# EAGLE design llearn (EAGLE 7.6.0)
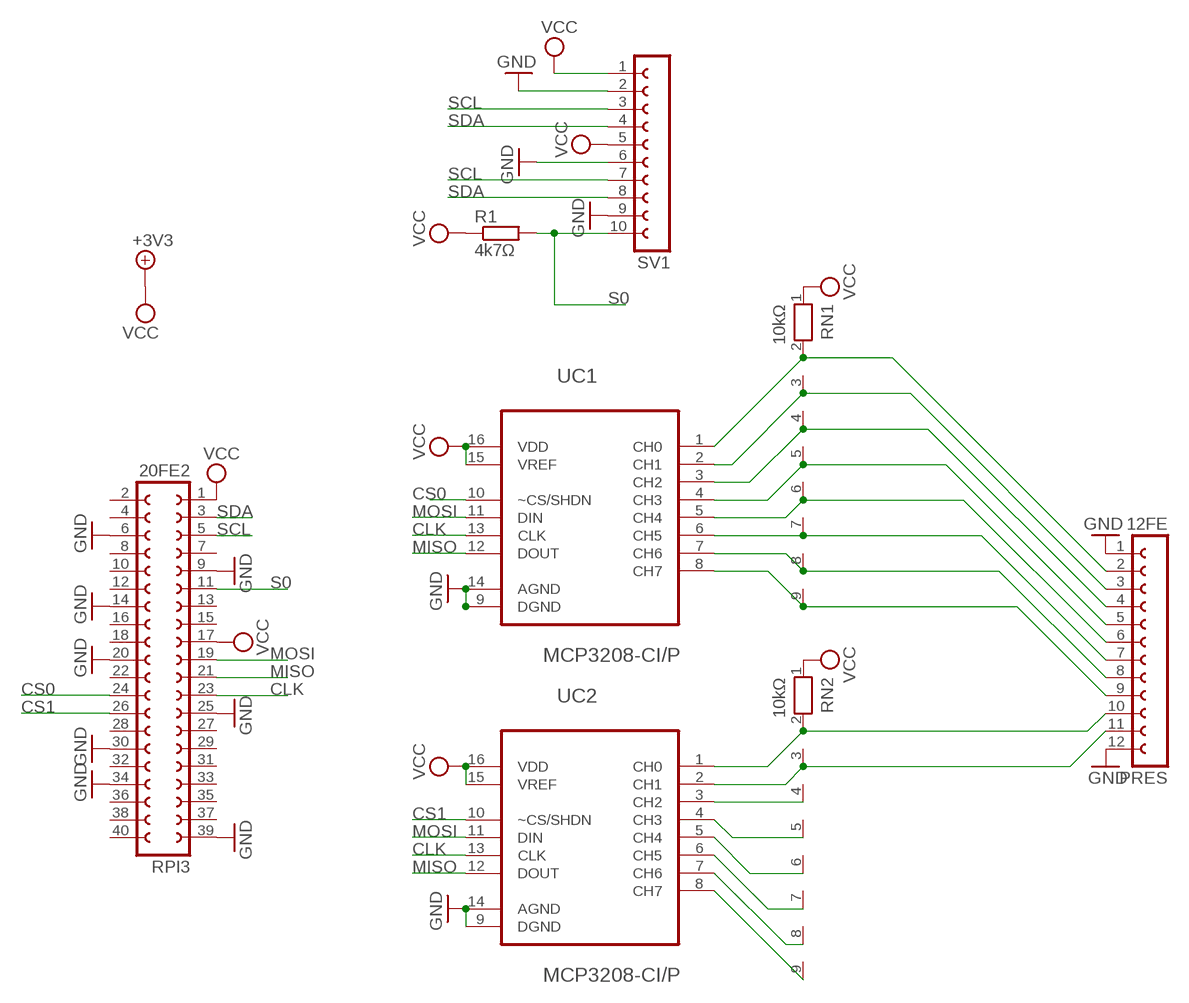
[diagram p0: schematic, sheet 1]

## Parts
PRES  12FE  FE12-1  [FE12]
R1  4k7Ω  R-EU_0207/10  [0207/10]
RN1  10kΩ  RN08  [RN-9]
RN2  10kΩ  RN08  [RN-9]
RPI3  20FE2  FE20-2  [FE20-2]
SV1  FE10-1  [FE10]
UC1  MCP3208-CI/P  [DIP254P762X432-16]
UC2  MCP3208-CI/P  [DIP254P762X432-16]

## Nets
CLK: RPI3.23 UC1.13(CLK) UC2.13(CLK)
CS0: RPI3.24 UC1.10(~CS/SHDN)
CS1: RPI3.26 UC2.10(~CS/SHDN)
GND: PRES.1 PRES.12 RPI3.6 RPI3.9 RPI3.14 RPI3.20 RPI3.25 RPI3.30 RPI3.34 RPI3.39 SV1.2 SV1.6 SV1.9 UC1.9(DGND) UC1.14(AGND) UC2.9(DGND) UC2.14(AGND)
MISO: RPI3.21 UC1.12(DOUT) UC2.12(DOUT)
MOSI: RPI3.19 UC1.11(DIN) UC2.11(DIN)
N$1: PRES.2 RN1.2 UC1.1(CH0)
N$2: PRES.3 RN1.3 UC1.2(CH1)
N$3: PRES.4 RN1.4 UC1.3(CH2)
N$4: PRES.5 RN1.5 UC1.4(CH3)
N$5: PRES.6 RN1.6 UC1.5(CH4)
N$6: PRES.7 RN1.7 UC1.6(CH5)
N$7: PRES.8 RN1.8 UC1.7(CH6)
N$8: PRES.9 RN1.9 UC1.8(CH7)
N$9: PRES.10 RN2.2 UC2.1(CH0)
N$10: PRES.11 RN2.3 UC2.2(CH1)
N$11: RN2.4 UC2.3(CH2)
N$12: RN2.5 UC2.4(CH3)
N$13: RN2.6 UC2.5(CH4)
N$14: RN2.7 UC2.6(CH5)
N$15: RN2.8 UC2.7(CH6)
N$16: RN2.9 UC2.8(CH7)
S0: R1.2 RPI3.11 SV1.10
SCL: RPI3.5 SV1.3 SV1.7
SDA: RPI3.3 SV1.4 SV1.8
VCC: R1.1 RN1.1 RN2.1 RPI3.1 RPI3.17 SV1.1 SV1.5 UC1.15(VREF) UC1.16(VDD) UC2.15(VREF) UC2.16(VDD) ; supply symbol labelled +3V3
Unconnected: RPI3.2 RPI3.4 RPI3.7 RPI3.8 RPI3.10 RPI3.12 RPI3.13 RPI3.15 RPI3.16 RPI3.18 RPI3.22 RPI3.27 RPI3.28 RPI3.29 RPI3.31 RPI3.32 RPI3.33 RPI3.35 RPI3.36 RPI3.37 RPI3.38 RPI3.40

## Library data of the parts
PRES = con-lsta:FE12-1: FEMALE HEADER; OC_FARNELL: unknown; OC_NEWARK: unknown
R1 = rcl:R-EU_: RESISTOR, European symbol
RN1 RN2 = resistor-net:RN08: RESISTOR NETWORK; OC_FARNELL: unknown; OC_NEWARK: unknown
RPI3 = con-lsta:FE20-2: FEMALE HEADER; OC_FARNELL: unknown; OC_NEWARK: unknown
SV1 = con-lsta:FE10-1: FEMALE HEADER; OC_FARNELL: unknown; OC_NEWARK: unknown
UC1 UC2 = Microchip_By_element14_Batch_1:MCP3208-CI/P: A/D Converters; MPN: MCP3208-CI/P; OC_FARNELL: 1084269; OC_NEWARK: 58K1815; PACKAGE: DIP-16; SUPPLIER: Microchip

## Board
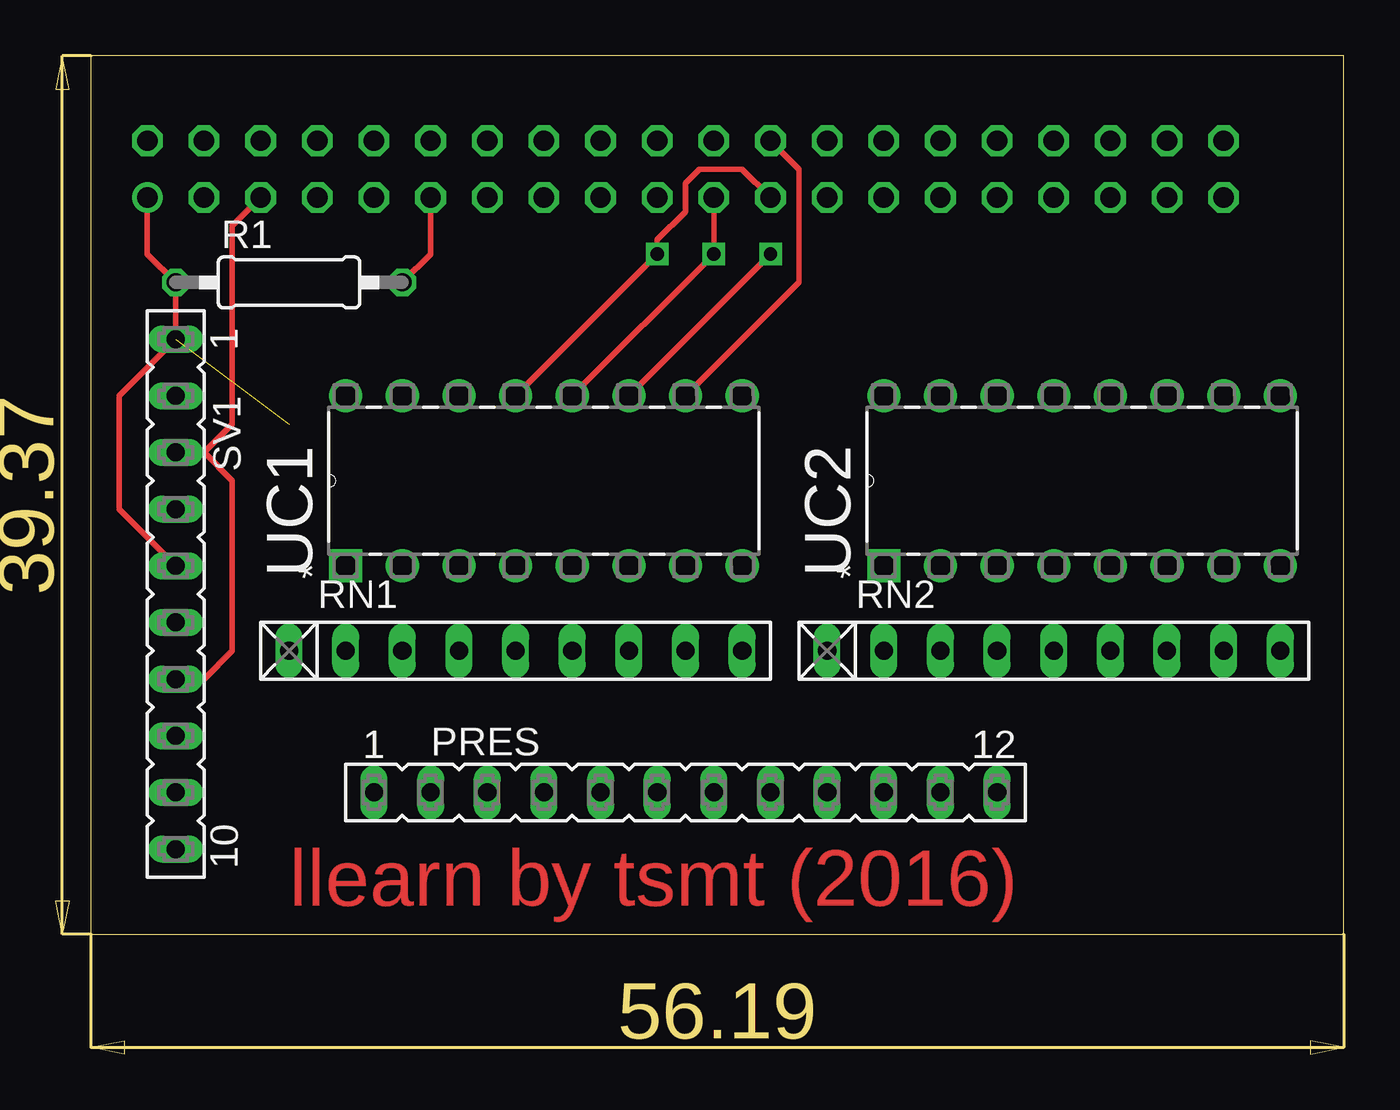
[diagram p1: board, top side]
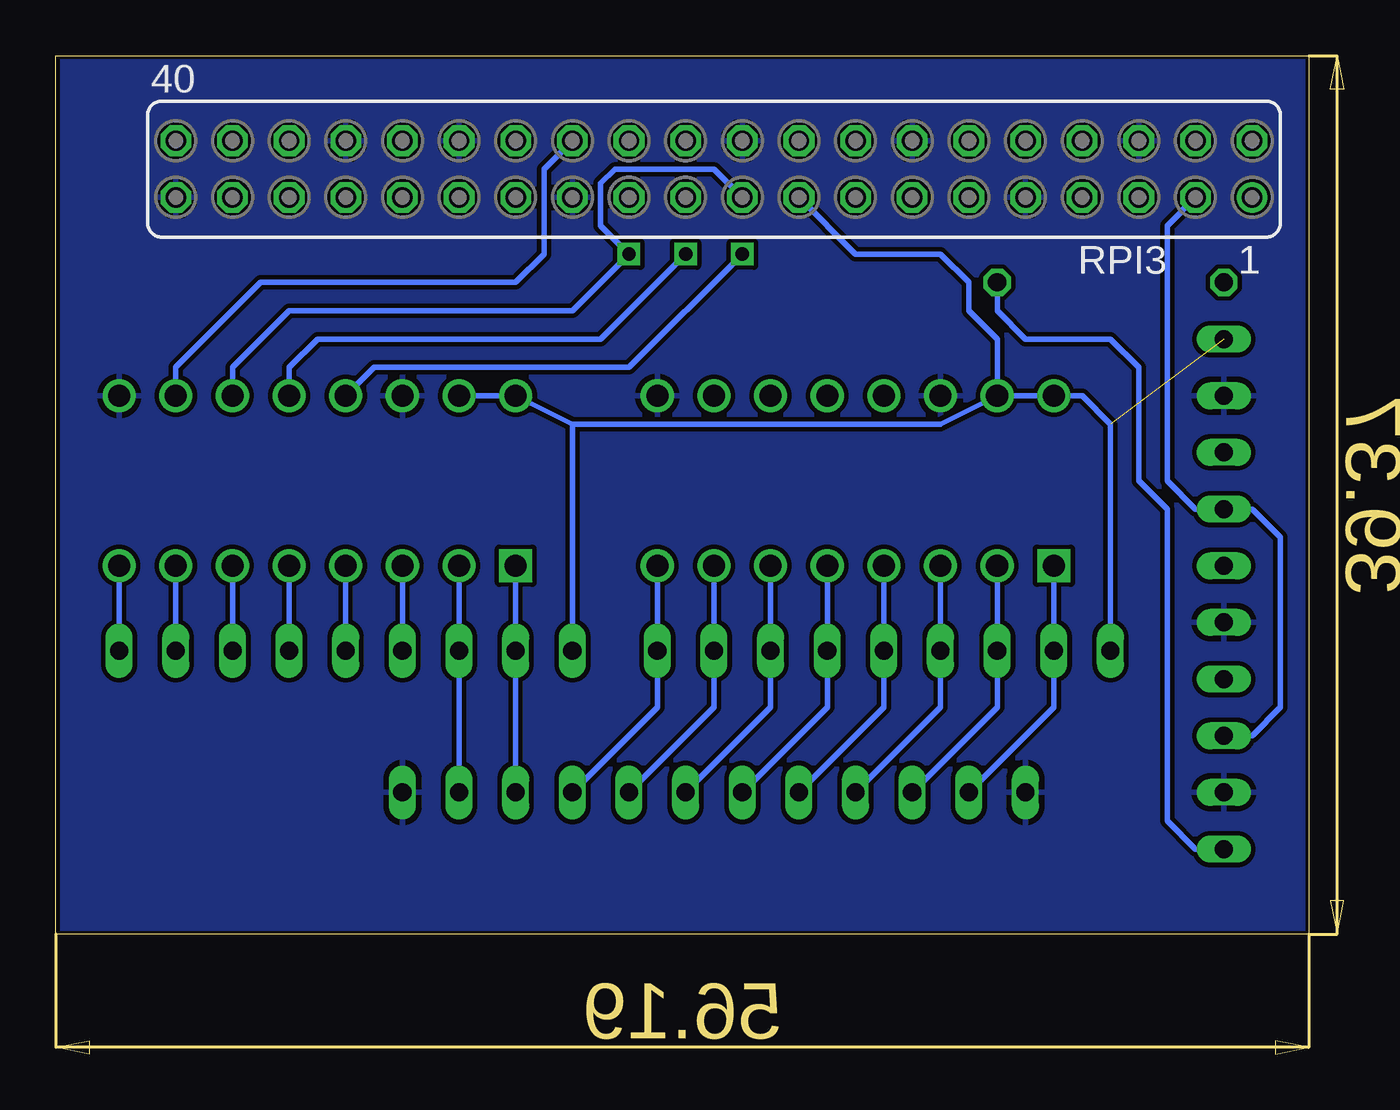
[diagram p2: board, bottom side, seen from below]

Size 57.76 x 44.75 mm. Coordinates in mm from the lower left corner, seen from the top.
Outline: 1.57,5.38 57.76,5.38 57.76,44.74 1.57,44.74 1.57,5.38
Copper layers (1*16): Top 0.035mm / dielectric 1.5mm / Bottom 0.035mm
Design rules "default *": minimum track width 0.2mm, minimum drill 0.3mm, track to track 8mil, track to pad 8mil, pad to pad 8mil, via to via 8mil, smd to smd 8mil, copper to edge 0.15mm, drill to drill 0.5mm, minimum pad ring 0.15mm, minimum via ring 8mil, stop-mask expansion 4mil, vias tented up to drill 0mil, thermal gap 10mil

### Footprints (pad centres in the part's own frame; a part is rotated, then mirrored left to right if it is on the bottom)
FE12 = drill 0.813 long: 1 -13.97,0; 2 -11.43,0; 3 -8.89,0; 4 -6.35,0; 5 -3.81,0; 6 -1.27,0; 7 1.27,0; 8 3.81,0; 9 6.35,0; 10 8.89,0; 11 11.43,0; 12 13.97,0
0207/10 = drill 0.813 octagon: 1 -5.08,0; 2 5.08,0
RN-9 = drill 0.813 long: 1 -10.16,0; 2 -7.62,0; 3 -5.08,0; 4 -2.54,0; 5 0,0; 6 2.54,0; 7 5.08,0; 8 7.62,0; 9 10.16,0
FE20-2 = drill 0.914: 1 -24.13,1.27 | drill 0.914 octagon: 2 -24.13,-1.27; 3 -21.59,1.27; 4 -21.59,-1.27; 5 -19.05,1.27; 6 -19.05,-1.27; 7 -16.51,1.27; 8 -16.51,-1.27; 9 -13.97,1.27; 10 -13.97,-1.27; 11 -11.43,1.27; 12 -11.43,-1.27; 13 -8.89,1.27; 14 -8.89,-1.27; 15 -6.35,1.27; 16 -6.35,-1.27; 17 -3.81,1.27; 18 -3.81,-1.27; 19 -1.27,1.27; 20 -1.27,-1.27; 21 1.27,1.27; 22 1.27,-1.27; 23 3.81,1.27; 24 3.81,-1.27; 25 6.35,1.27; 26 6.35,-1.27; 27 8.89,1.27; 28 8.89,-1.27; 29 11.43,1.27; 30 11.43,-1.27; 31 13.97,1.27; 32 13.97,-1.27; 33 16.51,1.27; 34 16.51,-1.27; 35 19.05,1.27; 36 19.05,-1.27; 37 21.59,1.27; 38 21.59,-1.27; 39 24.13,1.27; 40 24.13,-1.27
FE10 = drill 0.813 long: 1 -11.43,0; 2 -8.89,0; 3 -6.35,0; 4 -3.81,0; 5 -1.27,0; 6 1.27,0; 7 3.81,0; 8 6.35,0; 9 8.89,0; 10 11.43,0
DIP254P762X432-16 = drill 0.991 square: 1 -7.62,17.78 | drill 0.991: 2 -7.62,15.24; 3 -7.62,12.7; 4 -7.62,10.16; 5 -7.62,7.62; 6 -7.62,5.08; 7 -7.62,2.54; 8 -7.62,0; 9 0,0; 10 0,2.54; 11 0,5.08; 12 0,7.62; 13 0,10.16; 14 0,12.7; 15 0,15.24; 16 0,17.78

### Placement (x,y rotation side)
PRES  28.24,11.73 0 top
R1  10.46,34.59 0 top
RN1  20.62,18.08 0 top
RN2  44.75,18.08 0 top
RPI3  28.24,39.67 180 bottom
SV1  5.38,20.62 270 top
UC1  30.78,29.51 90 top
UC2  54.91,29.51 90 top

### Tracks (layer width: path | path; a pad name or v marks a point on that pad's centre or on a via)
CLK  (via drill 0.6)
  Top 0.254: RPI3.23 30.78,39.67 28.88,39.67 28.24,39.04 28.24,37.77 26.97,36.49 v26.97,35.86 UC1.13
  Bottom 0.254: v26.97,35.86 32.05,30.78 43.48,30.78 UC2.13
CS0
  Top 0.254: RPI3.24 33.32,39.67 33.32,34.59 UC1.10
CS1
  Bottom 0.254: RPI3.26 35.86,39.67 35.86,35.86 37.13,34.59 48.56,34.59 52.37,30.78 UC2.10
GND
  pour Bottom: 1.57,44.75 1.57,5.38 57.45,5.38 57.45,44.75
MISO  (via drill 0.6)
  Top 0.254: RPI3.21 v29.51,35.86 UC1.12
  Bottom 0.254: v29.51,35.86 33.32,32.05 46.02,32.05 47.29,30.78 UC2.12
MOSI  (via drill 0.6)
  Top 0.254: UC1.11 v32.05,35.86
  Bottom 0.254: RPI3.19 28.24,39.67 32.68,39.67 33.32,39.04 33.32,37.13 v32.05,35.86 34.59,33.32 47.29,33.32 49.83,30.78 UC2.11
N$1
  Bottom 0.254: UC1.1 RN1.2 13,15.54 PRES.2
N$2
  Bottom 0.254: UC1.2 RN1.3 15.54,15.54 PRES.3
N$3
  Bottom 0.254: UC1.3 RN1.4 18.08,15.54 PRES.4
N$4
  Bottom 0.254: UC1.4 RN1.5 20.62,15.54 PRES.5
N$5
  Bottom 0.254: UC1.5 RN1.6 23.16,15.54 PRES.6
N$6
  Bottom 0.254: UC1.6 RN1.7 25.7,15.54 PRES.7
N$7
  Bottom 0.254: UC1.7 RN1.8 28.24,15.54 PRES.8
N$8
  Bottom 0.254: UC1.8 RN1.9 30.78,15.54 PRES.9
N$9
  Bottom 0.254: UC2.1 RN2.2 PRES.10
N$10
  Bottom 0.254: UC2.2 RN2.3 PRES.11
N$11
  Bottom 0.254: UC2.3 RN2.4
N$12
  Bottom 0.254: UC2.4 RN2.5
N$13
  Bottom 0.254: UC2.5 RN2.6
N$14
  Bottom 0.254: UC2.6 RN2.7
N$15
  Bottom 0.254: UC2.7 RN2.8
N$16
  Bottom 0.254: UC2.8 RN2.9
S0
  Top 0.254: RPI3.11 16.81,35.86 R1.2
  Bottom 0.254: R1.2 15.54,33.32 14.27,32.05 10.46,32.05 9.19,30.78 9.19,25.7 7.92,24.43 7.92,10.46 6.65,9.19 SV1.10
SCL
  Top 0.254: 6.65,26.97 7.92,25.7 7.92,18.08 6.65,16.81 SV1.7 | SV1.3 6.65,26.97 | 6.65,26.97 7.92,28.24 7.92,37.13 RPI3.5
SDA
  Bottom 0.254: RPI3.3 7.92,37.13 7.92,25.7 6.65,24.43 SV1.4 4.11,24.43 2.84,23.16 2.84,15.54 4.11,14.27 SV1.8
VCC  (1 unrouted)
  Top 0.254: RPI3.1 4.11,35.86 R1.1 SV1.1 2.84,29.51 2.84,24.43 SV1.5
  Bottom 0.254: RPI3.17 21.89,35.86 18.08,35.86 16.81,34.59 16.81,33.32 15.54,32.05 UC1.15 | UC1.15 UC1.16 11.73,29.51 10.46,28.24 RN1.1 | UC1.15 18.08,28.24 34.59,28.24 | 34.59,28.24 UC2.16 UC2.15 | RN2.1 34.59,28.24

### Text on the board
Top: llearn by tsmt (2016)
